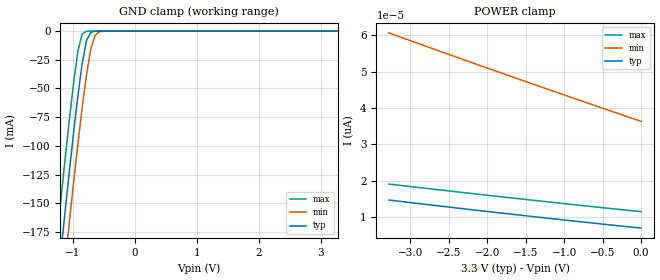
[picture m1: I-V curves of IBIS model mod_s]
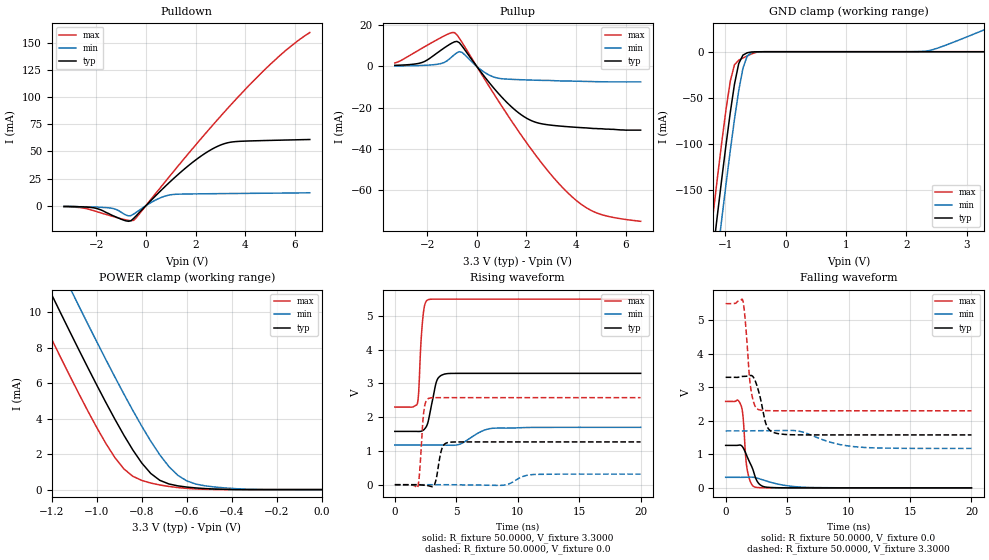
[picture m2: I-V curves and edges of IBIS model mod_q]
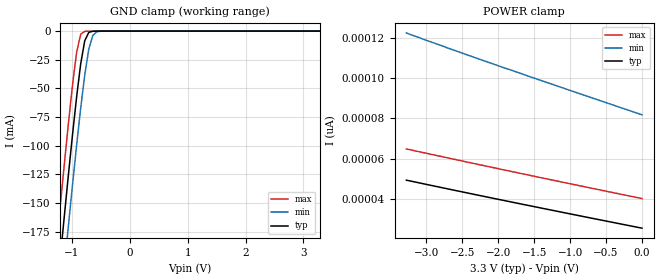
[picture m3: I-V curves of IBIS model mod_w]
| IBIS (I/O, Buffer, Information, Specification) Model, officially
| electronic behavioral standard for Buffer structures of digital pins.
[IBIS ver]  4.0
[File name] m95xxx_tssop8.ibs
[File Rev]  16
[Date]   27 June 2013
[Source]   CAD & Design Services (Catania) - STMicroelectronics
[Notes]
   (Note1)  This IBIS model includes the SO8 ceramic package parasitic data
   (Note2)  This IBIS model considers: VCC= 3.30(TYP), 1.70(MIN), 5.50(MAX)
   (Note3)  This IBIS model has some Notes about the non-monotonicity
   of the I-V curves, but they are not indicative of problems
   inside the model;
[Copyright] (c) 2013 STMicroelectronics
|   Component M95XXX
[Component] M95XXX
[Manufacturer] STMicroelectronics
[Package]
| variable   typ   min   max
R_pkg   0.0   0.0   0.0
L_pkg   0.0H   0.0H   0.0H
C_pkg   0.0F   0.0F   0.0F
[Pin]   signal_name   model_name   R_pin   L_pin   C_pin
1   SN   mod_s   NA   NA   NA
2   Q   mod_q   NA   NA   NA
3   WN   mod_w   NA   NA   NA
4   GND   GND   NA   NA   NA
5   D   mod_s   NA   NA   NA
6   C   mod_s   NA   NA   NA
7   HOLDN   mod_h   NA   NA   NA
8   VCC   POWER   NA   NA   NA
[Package Model]  182696_TSSOP8
[Define Package Model]  182696_TSSOP8
[Manufacturer]  STMicroelectronics
[OEM]  STMicroelectronics
[Description]  8 pin TSSOP package
[Number Of Pins]  8
[Pin Numbers]
|Pin Num   Terminal Name
1   | net1
2   | net2
3   | net3
4   | net4_GND
5   | net5
6   | net6
7   | net7
8   | net8_VDD
[Model Data]
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[End Model Data]
[End Package Model]
| Models and submodels in the file (4): mod_s (Input), mod_q (I/O), mod_w (Input), mod_h (Input)
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|   Model mod_s
[Model]   mod_s
Model_type Input
Vinl   =   1.00V
Vinh   =   2.30V
C_comp   2.119pF   2.024pF   2.323pF
[Temperature Range]  25.0000   85.0000   -40.0000
[Voltage Range]   3.3000V   1.7000V   5.5000V
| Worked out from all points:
|   GND clamp passes 1 mA (typ) near -0.70 V on its own axis
[GND_clamp]
|Voltage   I(typ)   I(min)   I(max)
-3.3V     -1.355A    -1.397A    -1.313A
-1.27V    -233mA     -277.9mA   -187.4mA
-1.2V     -196.1mA   -241mA     -150.5mA
-1.13V    -159.7mA   -204.5mA   -114.2mA
-1.06V    -124.1mA   -168.5mA   -79.16mA
-920mV    -57.12mA   -99.32mA   -18.15mA
-850mV    -28.51mA   -67.14mA   -2.609mA
-780mV    -8.357mA   -38.23mA   -131.1uA
-710mV    -1.089mA   -15.64mA   -5.451uA
-640mV    -95.71uA   -3.67mA    -224.5nA
-570mV    -7.943uA   -542uA     -9.245nA
3.28V     6.871pA    47.88pA    6.69pA
[POWER_clamp]
|Voltage   I(typ)   I(min)   I(max)
-3.28V    14.67pA    60.69pA    19.06pA
-1.76V    10.93pA    49.21pA    15.42pA
-880mV    8.889pA    42.72pA    13.4pA
0V        6.915pA    36.33pA    11.44pA
|   Model mod_q
[Model]   mod_q
Model_type I/O
Polarity   Non-Inverting
Enable   Active-Low
Vinl   =   1.00V
Vinh   =   2.30V
Vmeas  =   1.65V
Cref   =   30pF
C_comp   2.925pF   2.547pF   3.358pF
[Temperature Range]  25.0000   85.0000   -40.0000
[Voltage Range]   3.3000V   1.7000V   5.5000V
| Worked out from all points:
|   slope of the pulldown table from 0 to 0.495 V, typ, clamps not added: 43.1 ohm
|   slope of the pullup table from 0 to 0.495 V, typ, clamps not added: 63.8 ohm
|   GND clamp passes 1 mA (typ) near -0.63 V on its own axis
|   POWER clamp passes 1 mA (typ) near -0.77 V on its own axis
|   rising waveform, R_fixture 50.0000, V_fixture 3.3000: 20-80 % time 570ps typ, 1.43ns min, 290ps max; typ from 1.58 V to 3.3 V
|   rising waveform, R_fixture 50.0000, V_fixture 0.0: 20-80 % time 373ps typ, 964ps min, 282ps max; typ from 0 V to 1.27 V
|   falling waveform, R_fixture 50.0000, V_fixture 0.0: 20-80 % time 831ps typ, 2.11ns min, 339ps max; typ from 1.27 V to 0 V
|   falling waveform, R_fixture 50.0000, V_fixture 3.3000: 20-80 % time 642ps typ, 2.65ns min, 427ps max; typ from 3.3 V to 1.58 V
[Pulldown]
|Voltage   I(typ)   I(min)   I(max)
-3.3V     -700uA     -700uA     -1mA
-2.1V     -2mA       -1.2mA     -4.6mA
-1.3V     -9.5mA     -2.7mA     -10.1mA
-800mV    -14.04mA   -8.71mA    -13.17mA
-500mV    -11.87mA   -7.868mA   -13.57mA
300mV     7.031mA    4.108mA    8.594mA
900mV     20.46mA    9.617mA    25.58mA
2V        42.09mA    10.87mA    55.9mA
2.9V      54.9mA     11.09mA    79.73mA
3.5V      58.86mA    11.22mA    95mA
5V        60.21mA    11.52mA    130.2mA
6.6V      61.03mA    11.87mA    159.7mA
[Pullup]
|Voltage   I(typ)   I(min)   I(max)
-3.3V     521uA      215uA      1.668mA
-2.2V     1.926mA    483uA      8.876mA
-1.4V     8.241mA    1.523mA    14.28mA
-900mV    11.94mA    5.725mA    16.46mA
-600mV    10.01mA    6.891mA    11.84mA
600mV     -9.31mA    -4.769mA   -11.65mA
1.7V      -22.71mA   -6.436mA   -31.85mA
2.4V      -27.28mA   -6.709mA   -43.63mA
3.5V      -29.17mA   -7.1mA     -59.47mA
4.2V      -29.77mA   -7.25mA    -66.98mA
4.8V      -30.2mA    -7.42mA    -71.12mA
6.6V      -31mA      -7.53mA    -75.33mA
[GND_clamp]
|Voltage   I(typ)   I(min)   I(max)
-3.3V     -1.448A    -1.489A    -1.412A
-1.27V    -253.9mA   -297.7mA   -213.5mA
-1.2V     -214.5mA   -258.4mA   -174.1mA
-1.13V    -175.7mA   -219.5mA   -135.4mA
-1.06V    -137.7mA   -181.2mA   -97.89mA
-920mV    -66.08mA   -107.5mA   -32.04mA
-850mV    -35.23mA   -73.21mA   -14.1mA
-780mV    -12.93mA   -42.32mA   -9.262mA
-710mV    -3.708mA   -18mA      -6.819mA
-640mV    -1.177mA   -4.777mA   -4.574mA
2.3V      55.03pA    487.9uA    -209.6pA
3.28V     249.7pA    23.57mA    -17.59pA
[POWER_clamp]
|Voltage   I(typ)   I(min)   I(max)
-3.28V    67.55mA    69.89mA    65.16mA
-1.32V    14.15mA    16.63mA    11.63mA
-1.28V    13.09mA    15.58mA    10.57mA
-1.2V     10.99mA    13.48mA    8.479mA
-1.12V    8.922mA    11.4mA     6.427mA
-1.08V    7.9mA      10.37mA    5.424mA
-960mV    4.924mA    7.344mA    2.612mA
-880mV    3.078mA    5.401mA    1.172mA
-760mV    906.8uA    2.725mA    369.2uA
-640mV    211.2uA    805.3uA    114.6uA
-480mV    34.78uA    150.4uA    8.134uA
0V        255.5pA    464.6pA    417.5pA
[Ramp]
| variable   typ   min   max
dV/dt_r  0.7610/0.4100n   0.1882/1.1464n   1.5474/0.3147n
dV/dt_f  1.0304/0.7213n   0.3145/2.9896n   1.9193/0.4691n
R_load = 50.0000
[Rising Waveform]
R_fixture= 50.0000
V_fixture= 3.3000
V_fixture_min= 1.7000
V_fixture_max= 5.5000
|time   V(typ)   V(min)   V(max)
0s        1.58V      1.176V     2.301V
1.84ns    1.579V     1.177V     2.411V
1.94ns    1.578V     1.177V     2.728V
2.12ns    1.584V     1.177V     4.179V
2.28ns    1.607V     1.177V     4.943V
2.72ns    1.885V     1.177V     5.483V
3.4ns     3.067V     1.176V     5.5V
4.04ns    3.28V      1.173V     5.5V
7.96ns    3.3V       1.673V     5.5V
20ns      3.3V       1.7V       5.5V
[Rising Waveform]
R_fixture= 50.0000
V_fixture= 0.0
V_fixture_min= 0.0
V_fixture_max= 0.0
|time   V(typ)   V(min)   V(max)
0s        9.25nV     48.36nV    13.54nV
1.86ns    -406.5uV   788.9nV    -76.85mV
2.02ns    -3.537mV   2.922uV    385.6mV
2.34ns    -14.07mV   4.757uV    2.113V
2.74ns    -31.94mV   9.963uV    2.556V
3.22ns    -1.452mV   34.95uV    2.579V
3.82ns    1.056V     121.4uV    2.58V
4.36ns    1.253V     183.2uV    2.58V
11.42ns   1.268V     305.6mV    2.58V
20ns      1.268V     313.9mV    2.58V
[Falling Waveform]
R_fixture= 50.0000
V_fixture= 0.0
V_fixture_min= 0.0
V_fixture_max= 0.0
|time   V(typ)   V(min)   V(max)
0s        1.268V     313.9mV    2.58V
1.26ns    1.268V     313.8mV    2.451V
1.42ns    1.199V     314.6mV    2.107V
1.62ns    1.045V     316.5mV    966.9mV
1.74ns    941mV      318mV      574.4mV
2.02ns    713mV      321.5mV    176.5mV
2.34ns    402.7mV    310.3mV    30.02mV
2.78ns    99.06mV    266.9mV    5.944mV
3.54ns    13.79mV    179.4mV    452.7uV
20ns      9.542nV    1.308uV    -7.115nV
[Falling Waveform]
R_fixture= 50.0000
V_fixture= 3.3000
V_fixture_min= 1.7000
V_fixture_max= 5.5000
|time   V(typ)   V(min)   V(max)
0s        3.3V       1.7V       5.5V
1.4ns     3.327V     1.699V     5.591V
1.6ns     3.329V     1.699V     4.975V
2.04ns    3.356V     1.702V     2.974V
2.32ns    3.262V     1.705V     2.506V
2.64ns    2.936V     1.706V     2.343V
3.32ns    1.869V     1.707V     2.305V
4.2ns     1.623V     1.709V     2.301V
10.46ns   1.58V      1.23V      2.301V
20ns      1.58V      1.176V     2.301V
|   Model mod_w
[Model]   mod_w
Model_type Input
Vinl   =   1.00V
Vinh   =   2.30V
C_comp   2.119pF   2.024pF   2.323pF
[Temperature Range]  25.0000   85.0000   -40.0000
[Voltage Range]   3.3000V   1.7000V   5.5000V
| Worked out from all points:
|   GND clamp passes 1 mA (typ) near -0.70 V on its own axis
[GND_clamp]
|Voltage   I(typ)   I(min)   I(max)
-3.3V     -1.356A    -1.398A    -1.314A
-1.27V    -233.3mA   -278.1mA   -187.7mA
-1.2V     -196.3mA   -241.2mA   -150.7mA
-1.13V    -159.9mA   -204.6mA   -114.5mA
-1.06V    -124.2mA   -168.7mA   -79.35mA
-920mV    -57.23mA   -99.42mA   -18.3mA
-850mV    -28.6mA    -67.22mA   -2.741mA
-780mV    -8.431mA   -38.29mA   -241.4uA
-710mV    -1.144mA   -15.69mA   -94.22uA
-640mV    -131.4uA   -3.698mA   -67.87uA
-570mV    -27.41uA   -558.2uA   -47.22uA
3.28V     25.49pA    101pA      24.34pA
[POWER_clamp]
|Voltage   I(typ)   I(min)   I(max)
-3.28V    49.42pA    122.4pA    64.89pA
-2.72V    45.22pA    115.1pA    60.57pA
-1.88V    39.04pA    104.6pA    54.2pA
0V        25.63pA    81.81pA    40.3pA
